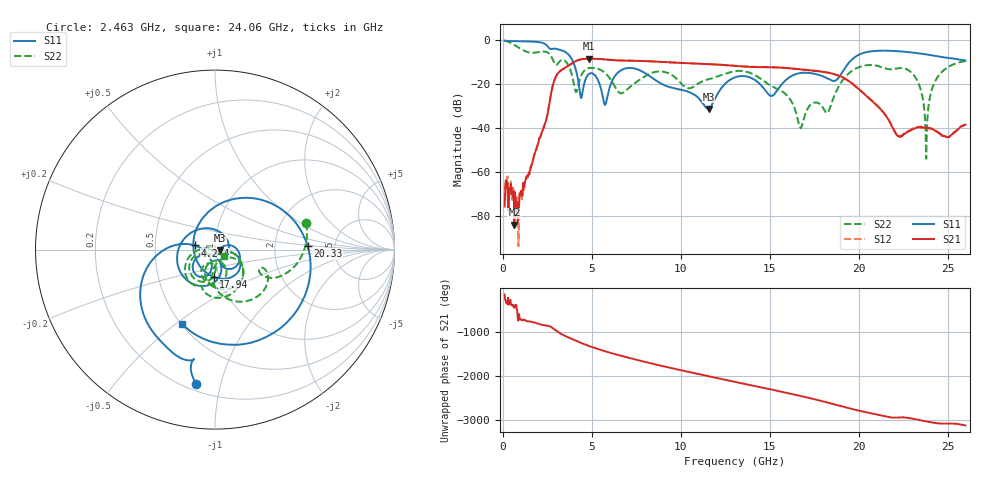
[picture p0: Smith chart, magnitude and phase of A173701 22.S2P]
!  2-Port S-parameters saved by WinCal
! VAR MeasName=S-Parameters (CALIBRATED_DATA) read from VNA (N5245A)
! VAR MeasDate=2017-6-7 10:29:50
! VAR NAME=A173701 22
! VAR FILENAME=A173701 22.S2P
! VAR DATE=2017-6-7 10:29:50
! VAR PHYS_PORTS=1,2
# Hz S DB R 50
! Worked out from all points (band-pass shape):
!   801 points, 100 MHz to 26 GHz, reference 50 ohm
!   highest |S21| = -8.53 dB at 4.859 GHz (marker M1); lowest = -83.8 dB at 650.4 MHz (marker M2)
!   |S21| within 3 dB of the highest: 3.712 GHz to 12.69 GHz (8.982 GHz wide, 109 % of centre); 12.69412 GHz to 12.73441 GHz (40.29 MHz wide, 0.317 % of centre)
!   lowest |S11| = -31.3 dB at 11.56 GHz (marker M3), VSWR 1.06, Z = 52.8 - j0.513 ohm
!   |S11| at or under -10 dB: 3.954 GHz to 19.49 GHz (15.54 GHz wide, 133 % of centre)
!   |S22| runs from -53.9 to -0.2 dB; largest |S21 - S12| = 0.0038
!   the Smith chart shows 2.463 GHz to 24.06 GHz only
!   S11 on the Smith chart (normalised r, x): 2.463 GHz: 0.24, -0.84; 4.244 GHz: 0.80, +0.04; 17.94 GHz: 0.94, -0.29; 20.33 GHz: 3.12, +0.17; 24.06 GHz: 0.51, -0.52
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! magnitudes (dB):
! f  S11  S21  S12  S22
! 100 MHz  -0.3  -75.6  -72.7  -0.2
! 650.4 MHz  -0.6  -83.8  -71.6  -2.3
! 2.463 GHz  -2.5  -35.4  -35.5  -5.5
! 3.014 GHz  -4.1  -16.2  -16.1  -11.4
! 4.244 GHz  -18.8  -9.1  -9.1  -20.4
! 4.438 GHz  -25.5  -8.7  -8.7  -15.7
! 4.859 GHz  -15.3  -8.5  -8.5  -12.7
! 5.733 GHz  -29.5  -8.8  -8.8  -14.9
! 6.802 GHz  -13.2  -9.4  -9.3  -23.8
! 8.744 GHz  -19.1  -9.9  -9.9  -14.3
! 11.56 GHz  -31.3  -11.0  -11.0  -17.9
! 13.05 GHz  -17.0  -11.8  -11.8  -14.2
! 15.12 GHz  -25.4  -12.4  -12.4  -21.0
! 16.74 GHz  -15.0  -13.4  -13.3  -40.1
! 17.39 GHz  -15.2  -13.9  -13.8  -28.8
! 17.94 GHz  -16.4  -14.4  -14.4  -30.0
! 20.33 GHz  -5.7  -24.6  -24.7  -11.6
! 21.69 GHz  -4.9  -36.5  -36.3  -13.3
! 23.15 GHz  -5.8  -40.2  -39.9  -16.5
! 23.8 GHz  -6.6  -39.8  -39.8  -53.9
! 24.06 GHz  -6.9  -40.3  -40.0  -24.1
! 26 GHz  -9.3  -38.5  -38.4  -9.7
